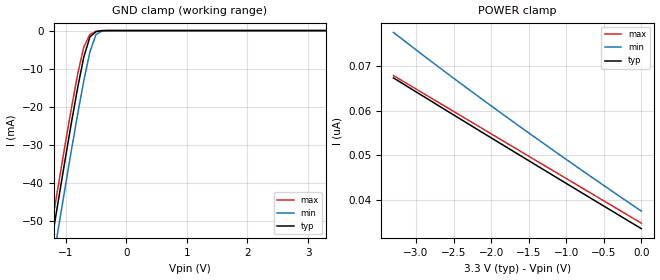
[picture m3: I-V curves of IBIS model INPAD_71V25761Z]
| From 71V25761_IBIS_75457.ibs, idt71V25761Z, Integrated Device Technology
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|   Model INPAD_71V25761Z
[Model]   INPAD_71V25761Z
Model_type   Input
Polarity   Non-Inverting
Vinl =  0.800V
Vinh =  2.000V
Vmeas =  1.500V
C_comp   1.56pF   1.56pF   1.56pF
[Temperature Range]   25.00   70.00   0.000
[Pullup Reference]   2.50V   2.37V   2.62V
[Pulldown Reference]   0.000V   0.000V   0.000V
[POWER Clamp Reference]   3.30V   3.13V   3.46V
[GND Clamp Reference]   0.000V   0.000V   0.000V
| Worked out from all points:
|   GND clamp passes 1 mA (typ) near -0.55 V on its own axis
[GND_clamp]
| voltage   I(typ)   I(min)   I(max)
-3.3V     -264mA     -271mA     -260mA
-1.3V     -62.17mA   -69.54mA   -58.12mA
-1.2V     -52.37mA   -59.74mA   -48.34mA
-1.1V     -42.67mA   -50.02mA   -38.65mA
-900mV    -23.78mA   -30.97mA   -19.92mA
-800mV    -14.87mA   -21.81mA   -11.29mA
-700mV    -6.924mA   -13.14mA   -4.258mA
-600mV    -1.699mA   -5.623mA   -1.019mA
-500mV    -276uA     -1.078mA   -189uA
-400mV    -20.39uA   -91.67uA   -9.996uA
-300mV    -1.424uA   -6.819uA   -531nA
3.3V      33.51nA    39.35nA    33.09nA
[POWER_clamp]
| voltage   I(typ)   I(min)   I(max)
-3.3V     67.41nA    77.64nA    67.95nA
-2.6V     60.13nA    68.62nA    60.89nA
-1.8V     51.89nA    58.68nA    52.83nA
-800mV    41.65nA    46.72nA    42.77nA
0V        33.51nA    37.45nA    34.74nA
